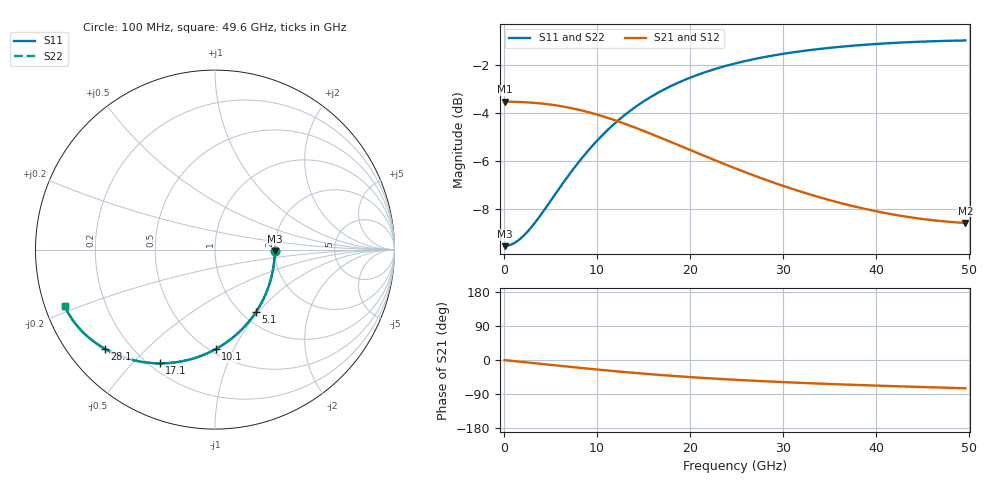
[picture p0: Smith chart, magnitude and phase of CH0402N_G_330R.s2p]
# GHz S RI R 330
! S-Parameters data
! Freq  reS11  imS11  reS21  imS21  reS12  imS12  reS22  imS22
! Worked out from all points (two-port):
!   100 points, 100 MHz to 49.6 GHz, reference 330 ohm
!   highest |S21| = -3.52 dB at 100 MHz (marker M1); lowest = -8.6 dB at 49.6 GHz (marker M2)
!   |S21| within 3 dB of the highest: start of sweep to 26.38 GHz
!   lowest |S11| = -9.5 dB at 100 MHz (marker M3), VSWR 2.00, Z = 660 - j11 ohm
!   |S11| at or under -10 dB: nowhere
!   |S22| runs from -9.5 to -1.0 dB; largest |S21 - S12| = 0
!   S11 on the Smith chart (normalised r, x): 100 MHz: 2.00, -0.03; 5.1 GHz: 1.16, -0.97; 10.1 GHz: 0.53, -0.85; 17.1 GHz: 0.24, -0.60; 28.1 GHz: 0.11, -0.38; 49.6 GHz: 0.06, -0.18
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0.1  0.3333 -0.00742  0.6667 -0.00294  0.6667 -0.00294  0.3333 -0.00742
1.1  0.328 -0.0813  0.6655 -0.0323  0.6655 -0.0323  0.328 -0.0813
2.6  0.3044 -0.1886  0.66 -0.0762  0.66 -0.0762  0.3044 -0.1886
3.6  0.279 -0.2557  0.6537 -0.105  0.6537 -0.105  0.279 -0.2557
5.1  0.2288 -0.3472  0.6405 -0.147  0.6405 -0.147  0.2288 -0.3472
7.1  0.1456 -0.4487  0.6158 -0.1996  0.6158 -0.1996  0.1456 -0.4487
8.6  0.0758 -0.5084  0.5926 -0.2353  0.5926 -0.2353  0.0758 -0.5084
10.1  0.00346 -0.5547  0.5663 -0.2671  0.5663 -0.2671  0.00346 -0.5547
11.6  -0.0687 -0.5887  0.5376 -0.2945  0.5376 -0.2945  -0.0687 -0.5887
13.1  -0.1389 -0.612  0.5077 -0.3175  0.5077 -0.3175  -0.1389 -0.612
14.6  -0.2057 -0.6262  0.4774 -0.3362  0.4774 -0.3362  -0.2057 -0.6262
16.6  -0.2883 -0.6337  0.4375 -0.3551  0.4375 -0.3551  -0.2883 -0.6337
17.1  -0.3077 -0.6339  0.4277 -0.3589  0.4277 -0.3589  -0.3077 -0.6339
19.1  -0.3802 -0.6294  0.3901 -0.3705  0.3901 -0.3705  -0.3802 -0.6294
21.1  -0.4445 -0.6183  0.3551 -0.3777  0.3551 -0.3777  -0.4445 -0.6183
23.1  -0.5013 -0.6026  0.3231 -0.3814  0.3231 -0.3814  -0.5013 -0.6026
25.1  -0.5512 -0.5838  0.2939 -0.3825  0.2939 -0.3825  -0.5512 -0.5838
28.1  -0.6148 -0.5522  0.2554 -0.3811  0.2554 -0.3811  -0.6148 -0.5522
33.1  -0.6964 -0.4957  0.2035 -0.3744  0.2035 -0.3744  -0.6964 -0.4957
37.1  -0.7451 -0.4504  0.1707 -0.3682  0.1707 -0.3682  -0.7451 -0.4504
41.6  -0.7868 -0.4009  0.1407 -0.3625  0.1407 -0.3625  -0.7868 -0.4009
49.6  -0.8364 -0.3164  0.0992 -0.3592  0.0992 -0.3592  -0.8364 -0.3164
